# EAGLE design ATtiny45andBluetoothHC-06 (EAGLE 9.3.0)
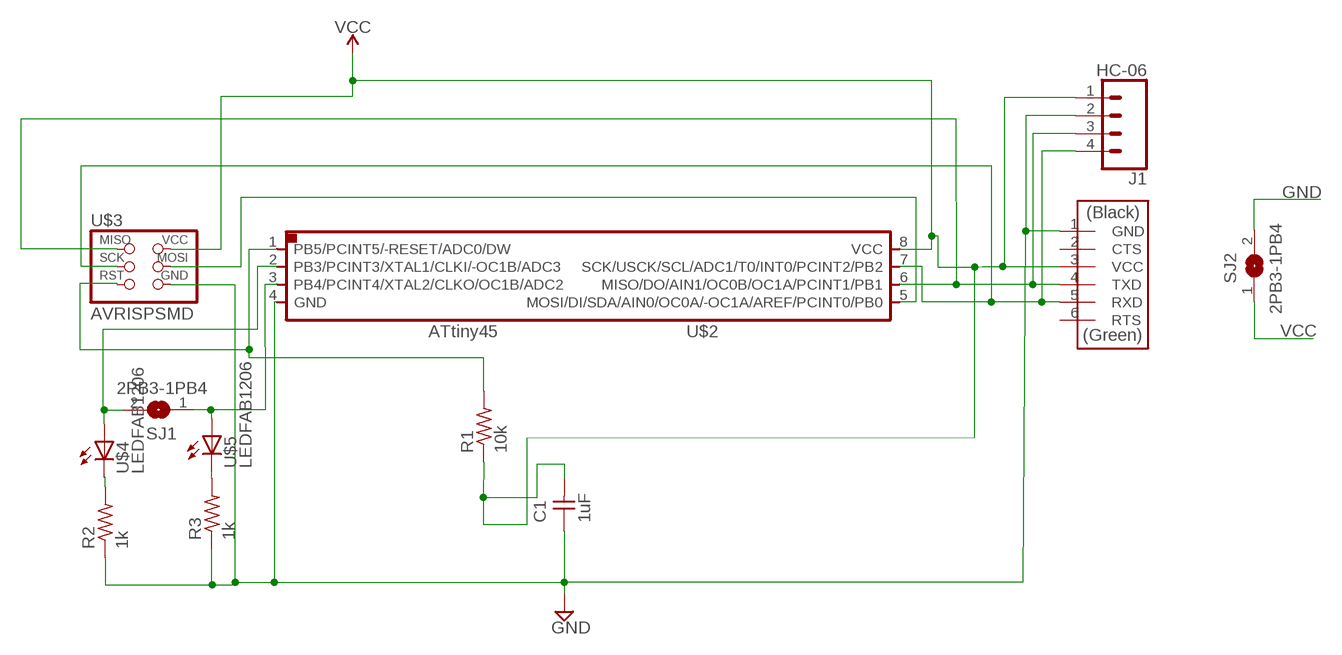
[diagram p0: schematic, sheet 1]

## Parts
C1  1uF  CAP-UNPOLARIZED  [C1206]
J1  HC-06  CONN_04SMD_RA_FEMALE  [1X04_SMD_RA_FEMALE]
R1  10k  RES-US1206  [R1206]
R2  1k  RES-US1206  [R1206]
R3  1k  RES-US1206  [R1206]
SJ1  2PB3-1PB4  SJW  [SJW]
SJ2  2PB3-1PB4  SJW  [SJW]
U$1  FTDI-SMD-HEADER  [1X06SMD]
U$2  ATTINY45SI  [SOIC8]
U$3  AVRISPSMD  [2X03SMD]
U$4  LEDFAB1206  [LED1206FAB]
U$5  LEDFAB1206  [LED1206FAB]

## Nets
GND: C1.1 J1.2 R2.1 R3.1 SJ2.2 U$1.1(GND) U$2.4(GND) U$3.6(GND)
N$1: J1.4 U$1.5(RXD) U$2.7(SCK/USCK/SCL/ADC1/T0/INT0/PCINT2/PB2) U$3.3(SCK)
N$2: R1.2 U$2.1(PB5/PCINT5/-RESET/ADC0/DW) U$3.5(RST)
N$3: SJ1.2 U$2.2(PB3/PCINT3/XTAL1/CLKI/-OC1B/ADC3) U$4.1(A)
N$4: U$2.5(MOSI/DI/SDA/AIN0/OC0A/-OC1A/AREF/PCINT0/PB0) U$3.4(MOSI)
N$5: J1.3 U$1.4(TXD) U$2.6(MISO/DO/AIN1/OC0B/OC1A/PCINT1/PB1) U$3.1(MISO)
N$6: SJ1.1 U$2.3(PB4/PCINT4/XTAL2/CLKO/OC1B/ADC2) U$5.1(A)
N$9: R2.2 U$4.2(C)
N$10: R3.2 U$5.2(C)
VCC: C1.2 J1.1 R1.1 SJ2.1 U$1.3(VCC) U$2.8(VCC) U$3.2(VCC)
Unconnected: U$1.2(CTS) U$1.6(RTS)

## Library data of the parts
C1 = fab:CAP-UNPOLARIZED
J1 = SparkFun-Connectors:CONN_04: Multi connection point. Often used as Generic Header-pin footprint for 0.1 inch spaced/style header connections On any of the 0.1 inch spaced packages, you can populate with these: Break Away Headers - Straight (PRT-00116) Break Away Male Headers - Right Angle (PRT-00553) Female Headers (PRT-00115)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; PROD_ID: CONN-12382
R1-R3 = fab:RES-US: Resistor (US Symbol)
SJ1 SJ2 = jumper:SJ: SMD solder JUMPER
U$1 = fab:FTDI-SMD-HEADER
U$2 = 01_fab:ATTINY45
U$3 = fab:AVRISP
U$4 U$5 = fab:LED: LED

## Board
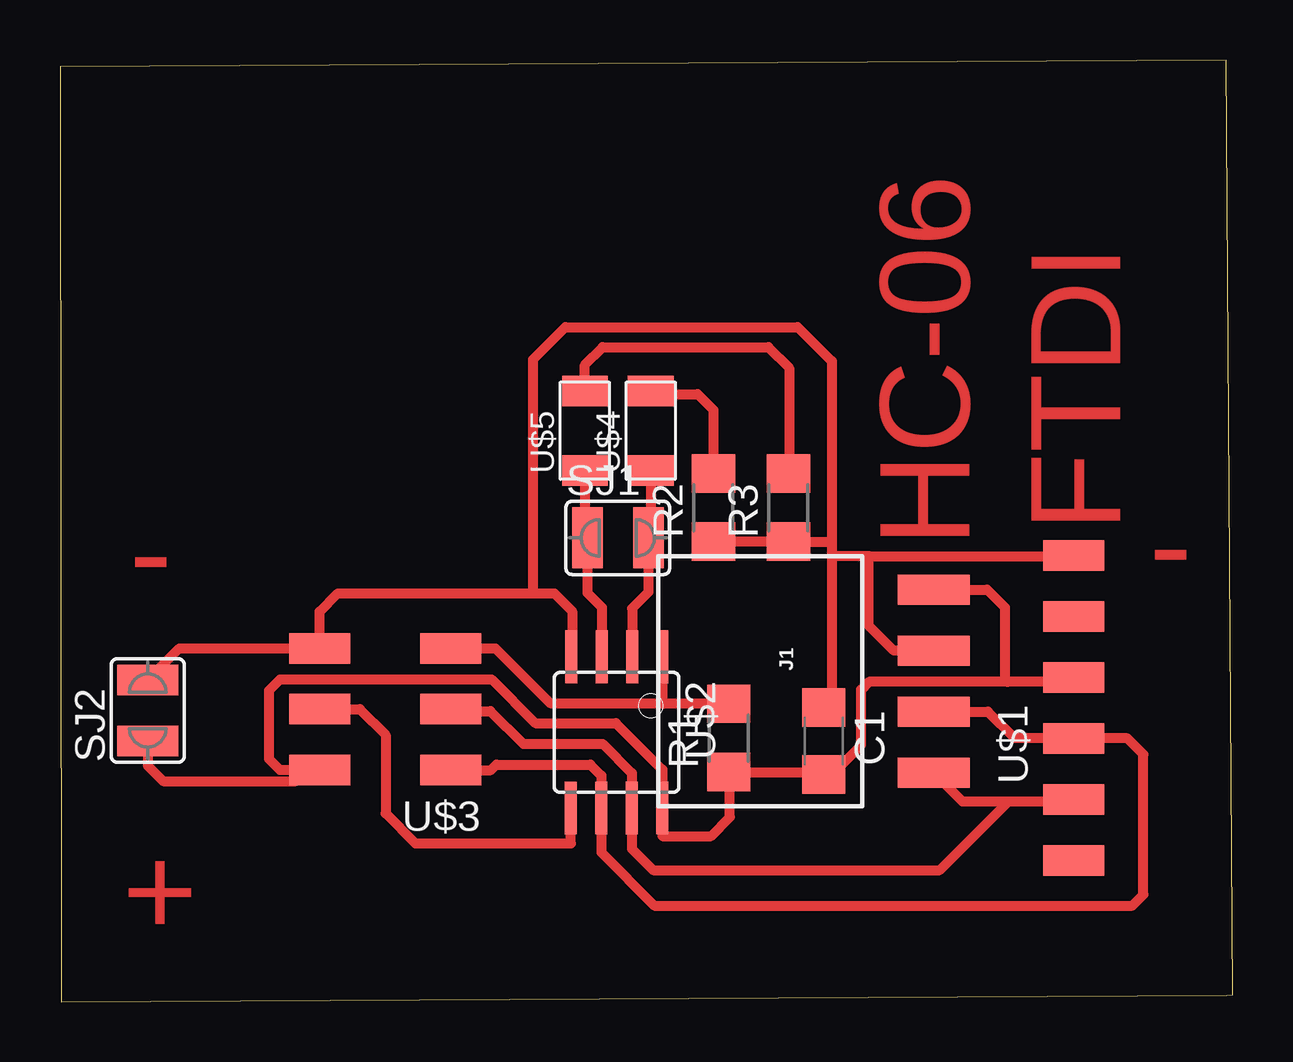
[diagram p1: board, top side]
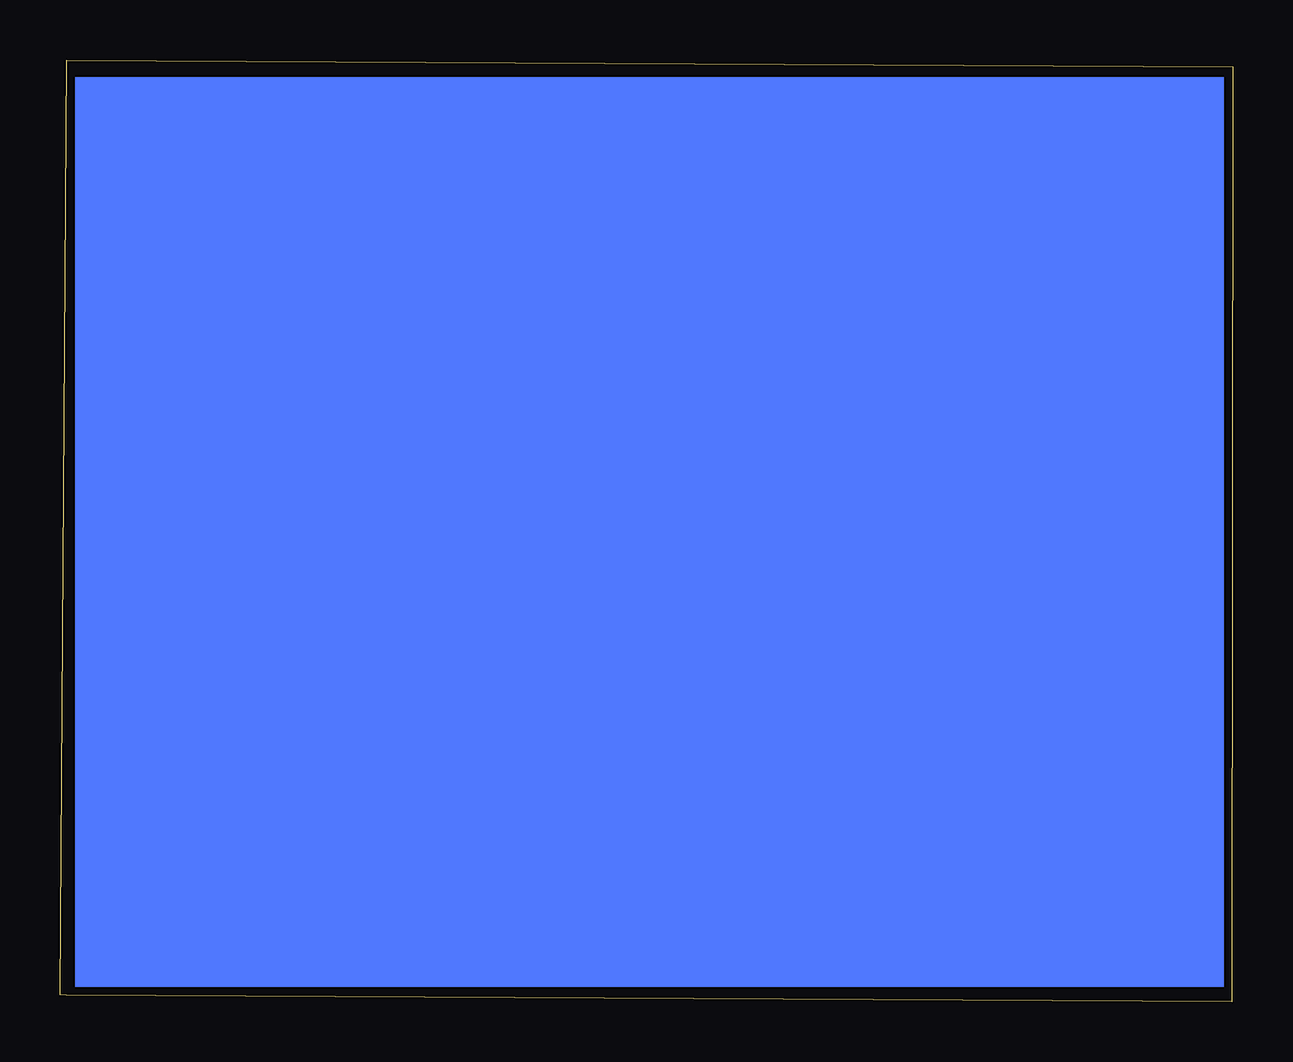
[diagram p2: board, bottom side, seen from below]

Size 48.87 x 39.24 mm. Coordinates in mm from the lower left corner, seen from the top.
Outline: 0,38.96 0.05,0 48.61,0.28 48.87,0.29 48.6,39.24 0,38.96
Copper layers (1*16): Top 0.035mm / dielectric 1.5mm / Bottom 0.035mm
Design rules "default": minimum track width 6mil, minimum drill 0.35mm, track to track 6mil, track to pad 6mil, pad to pad 6mil, via to via 6mil, smd to smd 6mil, copper to edge 40mil, drill to drill 6mil, minimum pad ring 10mil, minimum via ring 8mil, stop-mask expansion 4mil, vias tented up to drill 0mil, thermal gap 10mil

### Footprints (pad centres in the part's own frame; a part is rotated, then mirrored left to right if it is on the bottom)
C1206 = smd 1.6 x 1.8: 1 -1.4,0; 2 1.4,0
1X04_SMD_RA_FEMALE = smd 1.25 x 3: 1 -3.81,7.225; 2 -1.27,7.225; 3 1.27,7.225; 4 3.81,7.225
R1206 = smd 1.6 x 1.803: 1 -1.422,0; 2 1.422,0
SJW = smd 1.27 x 2.54: 1 -1.27,0; 2 1.27,0
1X06SMD = smd 2.54 x 1.27: 1 0,6.35; 2 0,3.81; 3 0,1.27; 4 0,-1.27; 5 0,-3.81; 6 0,-6.35
SOIC8 = smd 0.5 x 2.2: 1 -1.905,-3.154; 2 -0.645,-3.154; 3 0.625,-3.154; 4 1.895,-3.154; 5 1.905,3.154; 6 0.635,3.154; 7 -0.635,3.154; 8 -1.905,3.154
2X03SMD = smd 2.54 x 1.27: 1 -2.54,2.54; 2 2.92,2.54; 3 -2.54,0; 4 2.92,0; 5 -2.54,-2.54; 6 2.92,-2.54
LED1206FAB = smd 1.27 x 1.905: 1 -1.651,0; 2 1.651,0

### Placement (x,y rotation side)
C1  31.83,10.87 270 top
J1  29.18,13.36 270 top
R1  27.86,11 90 top
R2  27.23,20.6 90 top
R3  30.35,20.6 90 top
SJ1  23.24,19.33 0 top
SJ2  3.66,12.14 90 top
U$1  42.24,12.24 0 top
U$2  23.19,11.23 180 top
U$3  13.74,12.19 180 top
U$4  24.61,23.8 90 top
U$5  21.87,23.8 90 top

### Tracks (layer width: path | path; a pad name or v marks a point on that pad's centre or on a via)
GND
  Top 0.406: 19.63,17.02 11.58,17.02 10.82,16.26 U$3.6 4.98,14.73 SJ2.2 | 19.63,17.02 20.6,17.02 21.34,16.28 21.34,14.42 U$2.4 | 19.63,17.02 19.71,17.09 19.71,26.77 21.06,28.12 30.73,28.12 32.16,26.7 32.16,19.2 | 32.16,19.2 32.16,18.44 | 32.16,18.44 32.16,12.6 C1.1 | 33.71,18.57 42.21,18.57 U$1.1 | J1.2 34.75,14.63 33.71,15.67 33.71,18.57 | R2.1 R3.1 32.13,19.18 32.16,19.2 | 33.71,18.57 32.28,18.57 32.16,18.44
N$1
  Top 0.406: 39.52,8.36 36.65,5.49 24.71,5.49 23.83,6.38 U$2.7 23.83,9.52 22.61,10.74 19.3,10.74 17.93,12.12 16.36,12.12 U$3.3 | 39.52,8.36 42.16,8.36 U$1.5 | J1.4 37.6,8.36 39.52,8.36
N$2
  Top 0.406: U$3.5 18.14,14.73 20.42,12.45 25.1,12.45 | U$2.1 25.1,12.45 | R1.2 25.12,12.42 25.1,12.45
N$3
  Top 0.406: U$2.2 23.84,16.39 24.51,17.07 SJ1.2 24.61,19.43 U$4.1
N$4
  Top 0.406: U$3.4 12.5,12.19 13.56,11.13 13.56,7.85 14.81,6.6 21.29,6.6 U$2.5
N$5
  Top 0.406: U$3.1 17.96,9.65 18.19,9.88 22.1,9.88 22.56,9.42 U$2.6 22.56,6.22 24.77,4.01 44.68,4.01 45.14,4.47 45.14,10.31 44.48,10.97 U$1.4 42.21,11 39.75,11 38.66,12.09 J1.3
N$6
  Top 0.406: U$2.3 22.58,14.4 22.58,16.43 21.97,17.04 SJ1.1 21.87,19.43 U$5.1
N$9
  Top 0.406: U$4.2 24.74,25.32 26.57,25.32 27.23,24.66 R2.2
N$10
  Top 0.406: U$5.2 21.87,26.54 22.61,27.28 29.51,27.28 30.38,26.42 30.38,22.05 R3.2
VCC
  Top 0.406: U$1.3 42.06,13.33 39.47,13.33 | 39.47,13.33 33.71,13.33 33.38,13 33.38,10.69 32.15,9.47 C1.2 31.72,9.58 R1.1 27.91,9.53 27.91,7.7 27.13,6.91 25.1,6.91 U$2.8 25.1,9.68 23.16,11.61 19.81,11.61 17.98,13.44 9.17,13.44 8.71,12.98 8.71,10.11 9.17,9.65 10.29,9.65 | U$3.2 10.29,9.65 | J1.1 38.63,17.17 39.37,16.43 39.37,13.44 39.47,13.33 | SJ2.1 3.66,9.83 4.29,9.19 9.83,9.19 10.29,9.65
(copper drawn outside any net)
  shapes: Bottom area x1

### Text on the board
Top: FTDI | HC-06 | - | - | +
